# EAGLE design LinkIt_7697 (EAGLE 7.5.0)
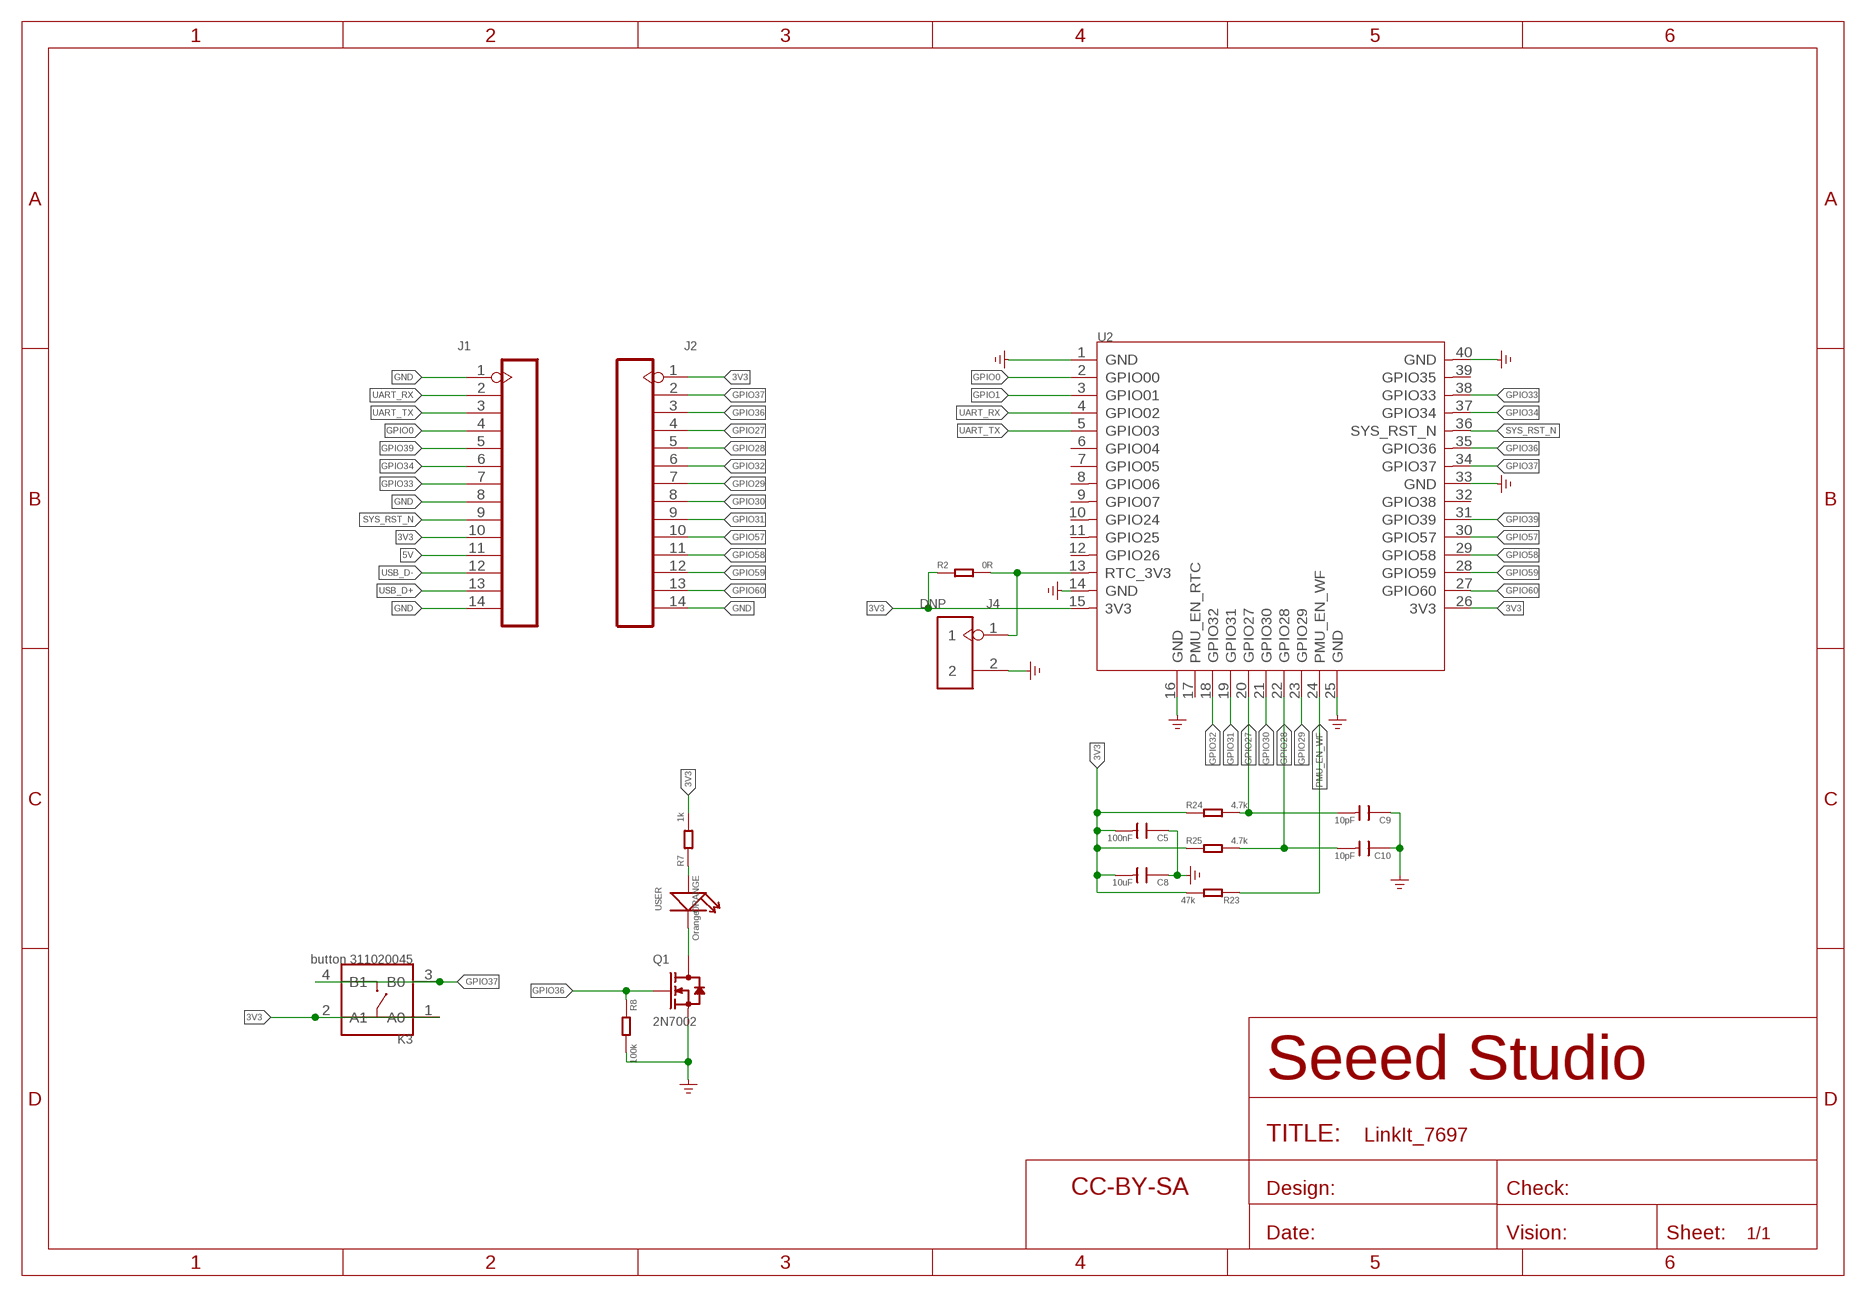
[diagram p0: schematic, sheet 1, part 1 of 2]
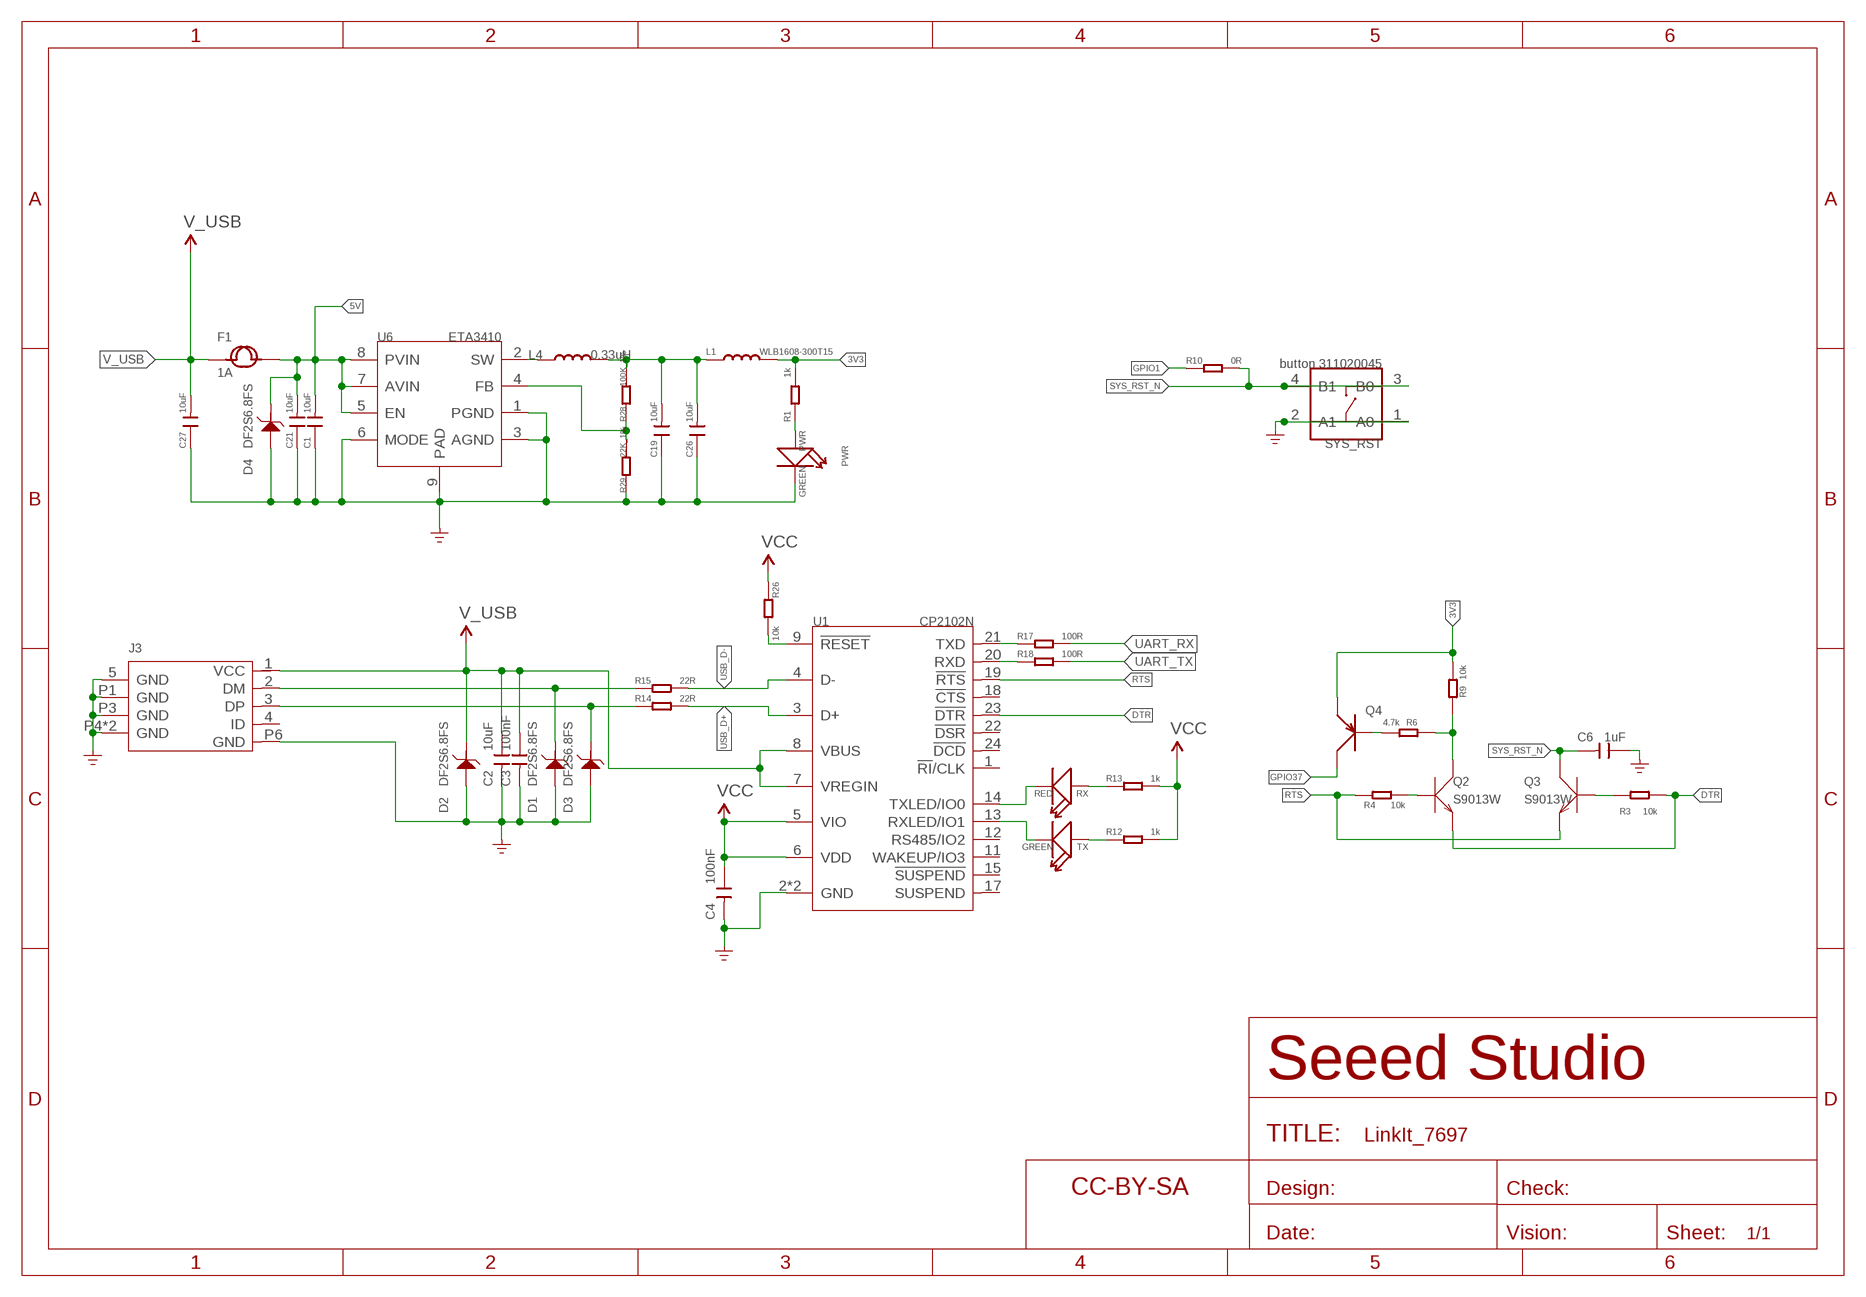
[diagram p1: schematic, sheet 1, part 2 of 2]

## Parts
C1  10uF  C-0402  [C0402]
C2  10uF  C-0402  [C0402]
C3  100nF  C-0402  [C0402]
C4  100nF  C-0402  [C0402]
C5  100nF  C-0402  [C0402]
C6  1uF  C-0402  [C0402]
C8  10uF  C-0402  [C0402]
C9  10pF  C-0402  [C0402]
C10  10pF  C-0402  [C0402]
C19  10uF  C-0402  [C0402]
C21  10uF  C-0402  [C0402]
C26  10uF  C-0402  [C0402]
C27  10uF  C-0402  [C0402]
D1  DF2S6.8FS  D-ESD-2P'DF2S6.8FS'  [SOD-923]
D2  DF2S6.8FS  D-ESD-2P'DF2S6.8FS'  [SOD-923]
D3  DF2S6.8FS  D-ESD-2P'DF2S6.8FS'  [SOD-923]
D4  DF2S6.8FS  D-ESD-2P'DF2S6.8FS'  [SOD-923]
F1  1A  FUSE'1206'  [F1206]
FR1  SEEEDSTUDIO-OPEN-SCH-FRAME  [SEEEDSTUDIO-PCB-FRAME]
FR2  SEEEDSTUDIO-OPEN-SCH-FRAME  [SEEEDSTUDIO-PCB-FRAME]
J1  HEADER-14P-2.54  [H14-2.54]
J2  HEADER-14P-2.54  [H14-2.54]
J3  MICRO-USB5+4P  [MICRO-USB5+5P-SMD-0.65-7.2X5.06MM]
J4  DNP  HEADER-2P-2.0  [H2-2.0-C55D32MIL]
K3  button 311020045  BUTTON-4P-4.5X3.2  [SW4P-SMD-4.5X3.2X2.5MM]
L1  WLB1608-300T15  L-0603  [L0603]
L4  0.33uH  L-MPM201610SR33_T  [L201610]
ORANGE  Orange  LED'0603'  [LED-0603]
PWR  GREEN  LED'0603'  [LED-0603]
Q1  2N7002  MOSFET-N'SI1304BDL'  [SOT-323]
Q2  S9013W  TRANSISTOR-NPN-SOT323  [SOT-323]
Q3  S9013W  TRANSISTOR-NPN-SOT323  [SOT-323]
Q4  TRANSISTOR-PNP  [SOT-323]
R1  1k  R-0402  [R0402]
R2  0R  R-0603  [R0603]
R3  10k  R-0402  [R0402]
R4  10k  R-0402  [R0402]
R6  4.7k  R-0402  [R0402]
R7  1k  R-0402  [R0402]
R8  100k  R-0402  [R0402]
R9  10k  R-0402  [R0402]
R10  0R  R-0402  [R0402]
R12  1k  R-0402  [R0402]
R13  1k  R-0402  [R0402]
R14  22R  R-0402  [R0402]
R15  22R  R-0402  [R0402]
R17  100R  R-0402  [R0402]
R18  100R  R-0402  [R0402]
R23  47k  R-0402  [R0402]
R24  4.7k  R-0402  [R0402]
R25  4.7k  R-0402  [R0402]
R26  10k  R-0402  [R0402]
R28  100K_1%  R-0402  [R0402]
R29  22K_1%  R-0402  [R0402]
RX  RED  LED'0603'  [LED-0603]
SYS_RST  button 311020045  BUTTON-4P-4.5X3.2  [SW4P-SMD-4.5X3.2X2.5MM]
TX  GREEN  LED'0603'  [LED-0603]
U1  CP2102N  CONVERTER-CP2102N(QFN24)  [QFN24G-0.5-4X4MM]
U2  MOUDLE-MT7697F  [MOUDLE40P-1.27-22X18MM]
U6  ETA3410  CONVERTER-ETA3410  [DFN8G-0.5-2X2MM]

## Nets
3V3: C5.2 C8.2 J1.10 J2.1 K3.1(A0) K3.2(A1) L1.2 Q4.2(E) R1.2 R2.1 R7.2 R9.1 R23.2 R24.1 R25.1 U2.15(3V3) U2.26(3V3)
5V: C1.2 C21.2 D4.1 F1.2 J1.11 U6.5(EN) U6.7(AVIN) U6.8(PVIN)
D-: D1.1 J3.2(DM) R15.1
DTR: Q2.2(E) R3.1 U1.23(!DTR!)
GND: C1.1 C2.2 C3.2 C4.2 C5.1 C6.1 C8.1 C9.1 C10.1 C19.1 C21.1 C26.1 C27.1 D1.2 D2.2 D3.2 D4.2 J1.1 J1.8 J1.14 J2.14 J3.5(GND) J3.P1(GND) J3.P3(GND) J3.P4(GND) J3.P5(GND) J3.P6(GND) J4.2 PWR.- Q1.2(S) R8.2 R29.1 SYS_RST.1(A0) SYS_RST.2(A1) U1.2(GND) U1.PAD(GND) U2.1(GND) U2.14(GND) U2.16(GND) U2.25(GND) U2.33(GND) U2.40(GND) U6.1(PGND) U6.3(AGND) U6.6(MODE) U6.9(PAD) ; supply symbol labelled GND_POWER
GPIO0: J1.4 U2.2(GPIO00)
GPIO1: R10.1 U2.3(GPIO01)
GPIO27: C9.2 J2.4 R24.2 U2.20(GPIO27)
GPIO28: C10.2 J2.5 R25.2 U2.22(GPIO28)
GPIO29: J2.7 U2.23(GPIO29)
GPIO30: J2.8 U2.21(GPIO30)
GPIO31: J2.9 U2.19(GPIO31)
GPIO32: J2.6 U2.18(GPIO32)
GPIO33: J1.7 U2.38(GPIO33)
GPIO34: J1.6 U2.37(GPIO34)
GPIO36: J2.3 Q1.1(G) R8.1 U2.35(GPIO36)
GPIO37: J2.2 K3.3(B0) K3.4(B1) Q4.3(C) U2.34(GPIO37)
GPIO39: J1.5 U2.31(GPIO39)
GPIO57: J2.10 U2.30(GPIO57)
GPIO58: J2.11 U2.29(GPIO58)
GPIO59: J2.12 U2.28(GPIO59)
GPIO60: J2.13 U2.27(GPIO60)
N$1: J4.1 R2.2 U2.13(RTC_3V3)
N$2: C19.2 C26.2 L1.1 L4.2 R28.2
N$3: D3.1 J3.3(DP) R14.1
N$4: PWR.+ R1.1
N$5: Q4.1(B) R6.1
N$6: ORANGE.+ R7.1
N$7: Q3.1(B) R3.2
N$8: ORANGE.- Q1.3(D)
N$9: Q2.1(B) R4.2
N$10: TX.- U1.13(RXLED/IO1)
N$11: Q2.3(C) R6.2 R9.2
N$13: RX.- U1.14(TXLED/IO0)
N$15: R26.2 U1.9(!RESET!)
N$17: R18.1 U1.20(RXD)
N$18: R17.1 U1.21(TXD)
N$29: L4.1 U6.2(SW)
N$32: R28.1 R29.2 U6.4(FB)
N$36: R12.1 TX.+
N$37: R13.1 RX.+
PMU_EN_WF: R23.1 U2.24(PMU_EN_WF)
RTS: Q3.2(E) R4.1 U1.19(!RTS!)
SYS_RST_N: C6.2 J1.9 Q3.3(C) R10.2 SYS_RST.3(B0) SYS_RST.4(B1) U2.36(SYS_RST_N)
UART_RX: J1.2 R17.2 U2.4(GPIO02)
UART_TX: J1.3 R18.2 U2.5(GPIO03)
USB_D+: J1.13 R14.2 U1.3(D+)
USB_D-: J1.12 R15.2 U1.4(D-)
V_USB: C2.1 C3.1 C27.2 D2.1 F1.1 J3.1(VCC) U1.7(VREGIN) U1.8(VBUS)
VCC: C4.1 R12.2 R13.2 R26.1 U1.5(VIO) U1.6(VDD)
Unconnected: J3.4(ID) U1.1(!RI!/CLK) U1.11(WAKEUP/IO3) U1.12(RS485/IO2) U1.15(!SUSPEND!) U1.17(SUSPEND) U1.18(!CTS!) U1.22(!DSR!) U1.24(!DCD!) U2.6(GPIO04) U2.7(GPIO05) U2.8(GPIO06) U2.9(GPIO07) U2.10(GPIO24) U2.11(GPIO25) U2.12(GPIO26) U2.17(PMU_EN_RTC) U2.32(GPIO38) U2.39(GPIO35)

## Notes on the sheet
- PWR
- USER

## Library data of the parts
C1-C6 C8-C10 C19 C21 C26 C27 = Discrete-small:C*: Ceramic Capacitors
D1-D4 = Discrete-new:D-ESD-2P: SOD-923:304060009;SOD-123:304060001
F1 = C-R-package test:FUSE
FR1 FR2 = moudle-new:SEEEDSTUDIO-OPEN-SCH-FRAME
J1 J2 = Connector-new:HEADER-14P: Header 14 Standard 14-pin 0.1" header. Use with straight break away headers (SKU : PRT-00116), right angle break away headers (PRT-00553), swiss pins (PRT-00743), machine pins (PRT-00117), and female headers (PRT-00115).
J3 = Connector-new:MICRO-USB5+4P: 5+4P-SMD-0.65-B:320010000;5+2P-SMD-0.65-AB:340032001;5+5P-SMD-0.65-7.2X5.06MM:320010050;
J4 = Connector-new:HEADER-2P
K3 SYS_RST = Discrete-new:BUTTON-4P: SW4-6.0X6.0X5.0MM:311020024;SW4-8.0X8.0X9.0MM:311020028;SW4-SMD-6.0X6.0X5.0MM:311020004;SW4-SMD-3.35X3.35X1.5MM:311020030;SW4-SMD-5.2X5.2X2.5MM:311020046
L1 = Discrete-small:L
L4 = Discrete-new:L
ORANGE PWR RX TX = Discrete-small:LED
Q1 = Discrete-new:MOSFET-N
Q2 Q3 = Discrete-new:TRANSISTOR-NPN: NPN audion
Q4 = Discrete-new:TRANSISTOR-PNP: PNP audion
R1-R4 R6-R10 R12-R15 R17 R18 R23-R26 R28 R29 = Discrete-small:R*
U1 = template:CONVERTER-CP2102N(QFN24)
U2 = template:MOUDLE-MT7697F
U6 = template:CONVERTER-ETA3410: 3MHZ 2A High Step-Down Converter in DFN2x2-8L Package

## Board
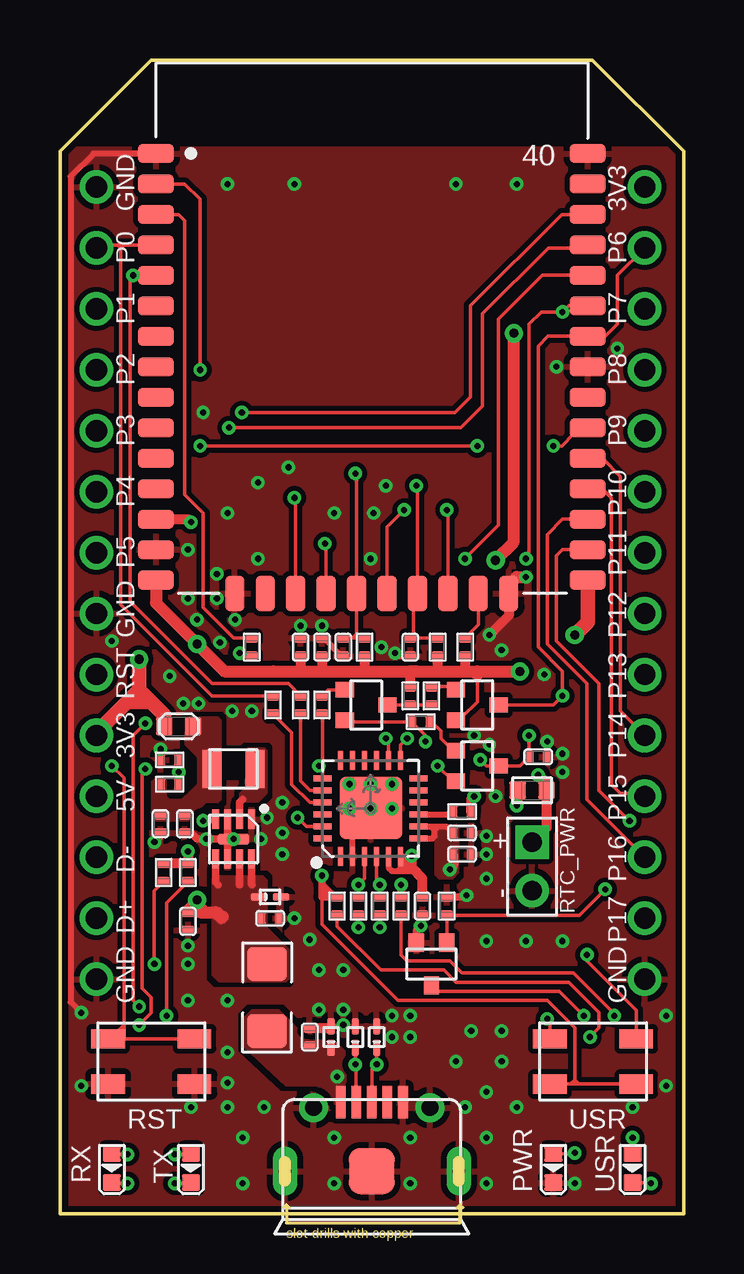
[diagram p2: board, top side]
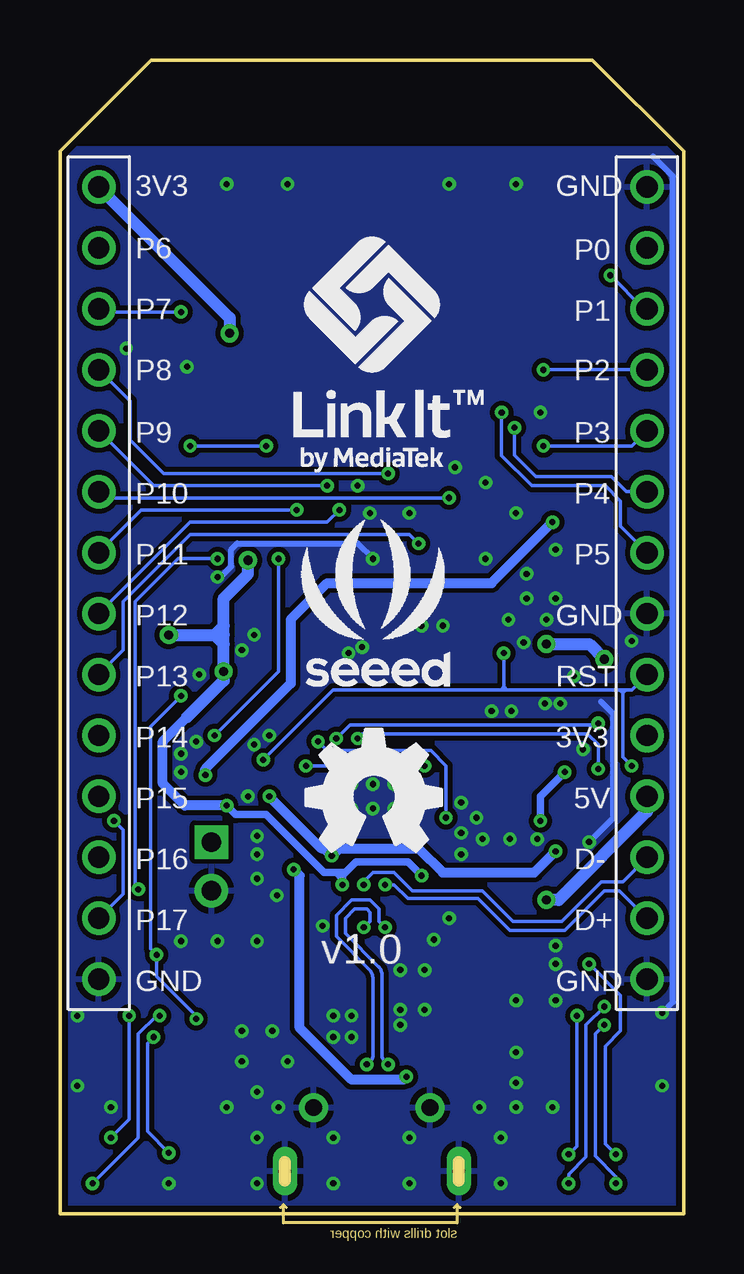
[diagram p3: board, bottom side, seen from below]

Size 26 x 48.09 mm. Coordinates in mm from the lower left corner, seen from the top.
Outline: 0,0 26,0 26,44.28 22.19,48.09 3.81,48.09 0,44.28 0,0
Copper layers (1*16): Top 0.035mm / dielectric 1.5mm / Bottom 0.035mm
Design rules "SeeedStudio_2layer_DRU_no_angle_20140221 *": minimum track width 1mil, minimum drill 10mil, track to track 6mil, track to pad 6mil, pad to pad 6mil, via to via 6mil, smd to smd 0mil, copper to edge 10mil, drill to drill 10mil, minimum pad ring 10mil, minimum via ring 6mil, stop-mask expansion 2mil, vias tented up to drill 25mil, thermal gap 10mil
tRestrict: area 0,44.7 to 26,48.3; area 7,18.3 to 7.5,19.3
bRestrict: area 0,44.7 to 26,48.3

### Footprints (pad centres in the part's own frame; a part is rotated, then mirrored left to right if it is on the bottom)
C0402 = smd 0.508 x 0.385: 1 0,0.383; 2 0,-0.383
SOD-923 = smd 0.7 x 0.3: 1 -0.45,0; 2 0.45,0
F1206 = smd 1.397 x 1.651: 1 -1.397,0; 2 1.397,0
H14-2.54 = drill 0.889 pad 1.397: 1 0,-16.51; 2 0,-13.97; 3 0,-11.43; 4 0,-8.89; 5 0,-6.35; 6 0,-3.81; 7 0,-1.27; 8 0,1.27; 9 0,3.81; 10 0,6.35; 11 0,8.89; 12 0,11.43; 13 0,13.97; 14 0,16.51
MICRO-USB5+5P-SMD-0.65-7.2X5.06MM = smd 0.4 x 1.35: 1 -1.3,2.875; 2 -0.65,2.875; 3 0,2.875; 4 0.65,2.875; 5 1.3,2.875 | smd 1.9 x 1.9: P1 0,0 | drill 0.508 pad 1.016 long: P3 -3.625,0; P4 3.625,0 | drill 0.7: P5 -2.425,2.65; P6 2.425,2.65
H2-2.0-C55D32MIL = drill 0.813 pad 1.397 square: 1 -1.016,0 | drill 0.813 pad 1.397: 2 1.016,0
SW4P-SMD-4.5X3.2X2.5MM = smd 1.4 x 0.8: 1 -1.8,-0.94; 2 1.8,-0.94; 3 1.8,0.94; 4 -1.8,0.94
L0603 = smd 0.762 x 0.696: 1 0,0.602; 2 0,-0.602
L201610 = smd 0.8 x 1.6: 1 -0.9,0; 2 0.9,0
LED-0603 = smd 0.696 x 0.762: + -0.602,0; - 0.602,0
SOT-323 = smd 0.635 x 0.762: 1 -0.635,-0.889; 2 0.635,-0.889; 3 0,0.889
R0402 = smd 0.508 x 0.385: 1 0,0.383; 2 0,-0.383
R0603 = smd 0.762 x 0.696: 1 0,0.602; 2 0,-0.602
QFN24G-0.5-4X4MM = smd 0.8 x 0.26: 1 -2,1.25; 2 -2,0.75; 3 -2,0.25; 4 -2,-0.25; 5 -2,-0.75; 6 -2,-1.25; 13 2,-1.25; 14 2,-0.75; 15 2,-0.25; 16 2,0.25; 17 2,0.75; 18 2,1.25 | smd 0.26 x 0.8: 7 -1.25,-2; 8 -0.75,-2; 9 -0.25,-2; 10 0.25,-2; 11 0.75,-2; 12 1.25,-2; 19 1.25,2; 20 0.75,2; 21 0.25,2; 22 -0.25,2; 23 -0.75,2; 24 -1.25,2 | smd 2.6 x 2.6: PAD 0.02,-0.01
MOUDLE40P-1.27-22X18MM = smd 1.5 x 0.8: 1 -9,8.89; 2 -9,7.62; 3 -9,6.35; 4 -9,5.08; 5 -9,3.81; 6 -9,2.54; 7 -9,1.27; 8 -9,0; 9 -9,-1.27; 10 -9,-2.54; 11 -9,-3.81; 12 -9,-5.08; 13 -9,-6.35; 14 -9,-7.62; 15 -9,-8.89; 26 9,-8.89; 27 9,-7.62; 28 9,-6.35; 29 9,-5.08; 30 9,-3.81; 31 9,-2.54; 32 9,-1.27; 33 9,0; 34 9,1.27; 35 9,2.54; 36 9,3.81; 37 9,5.08; 38 9,6.35; 39 9,7.62; 40 9,8.89 | smd 0.8 x 1.5: 16 -5.715,-9.45; 17 -4.445,-9.45; 18 -3.175,-9.45; 19 -1.905,-9.45; 20 -0.635,-9.45; 21 0.635,-9.45; 22 1.905,-9.45; 23 3.175,-9.45; 24 4.445,-9.45; 25 5.715,-9.45
DFN8G-0.5-2X2MM = smd 0.8 x 0.3: 1 -0.827,0.75; 2 -0.827,0.25; 3 -0.827,-0.25; 4 -0.827,-0.75; 5 0.827,-0.75; 6 0.827,-0.25; 7 0.827,0.25; 8 0.827,0.75 | smd 0.45 x 1.3: 9 0,0

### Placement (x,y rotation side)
C1  5.33,12.19 180 top
C2  16.76,14.99 90 top
C3  16.76,15.88 90 top
C4  15.11,12.83 0 top
C5  10.03,23.62 0 top
C6  19.94,19.05 270 top
C8  10.92,23.62 0 top
C9  11.81,23.62 180 top
C10  14.61,23.62 180 top
C19  5.21,16.26 180 top
C21  8.76,12.32 270 top
C26  4.19,16.26 180 top
C27  10.41,7.37 0 top
D1  12.32,7.37 90 top
D2  11.3,7.37 90 top
D3  13.21,7.37 90 top
D4  8.76,13.21 0 top
F1  8.64,9.02 90 top
FR1  not placed on the board
FR2  not placed on the board
J1  1.52,26.29 180 bottom
J2  24.38,26.29 180 bottom
J3  13,1.78 0 top
J4  19.68,14.48 270 top
K3  22.23,6.35 0 top
L1  4.95,20.32 270 top
L4  7.24,18.54 180 top
ORANGE  23.88,1.91 270 top
PWR  20.57,1.91 270 top
Q1  15.49,10.41 180 top
Q2  12.76,21.21 270 top
Q3  17.4,18.67 270 top
Q4  17.4,21.21 270 top
R1  11.56,12.83 180 top
R2  19.68,17.65 90 top
R3  15.05,20.51 90 top
R4  10.92,21.21 180 top
R6  15.49,21.59 0 top
R7  14.22,12.83 180 top
R8  16.13,12.83 180 top
R9  14.61,21.59 0 top
R10  8,23.62 0 top
R12  5.33,14.22 180 top
R13  4.32,14.22 180 top
R14  12.45,12.83 180 top
R15  13.34,12.83 180 top
R17  8.89,21.21 180 top
R18  10.03,21.21 180 top
R23  16.89,23.62 0 top
R24  12.7,23.62 180 top
R25  15.75,23.62 180 top
R26  16.76,16.76 270 top
R28  4.57,17.91 270 top
R29  4.57,18.92 90 top
RX  2.16,1.91 270 top
SYS_RST  3.81,6.35 0 top
TX  5.46,1.91 270 top
U1  12.95,16.89 90 top
U2  13,35.31 0 top
U6  7.24,15.62 270 top
U$1  [OSHW_FILLX200_NOTEXT_TNAME]  15.75,15.11 0 bottom
U$3  [SEEED-SILK-TNAME-280*268MIL]  12.95,25.65 0 bottom

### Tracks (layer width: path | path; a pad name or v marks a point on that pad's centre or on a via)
3V3  (via drill 0.25 pad 0.51, 0.38 pad 0.76)
  Top 0.152: K3.2 21.64,5.41 | 21.64,5.41 21.46,5.41 | 21.46,5.41 21.29,5.41 | 21.29,5.41 K3.1 | 21.46,5.59 21.46,7.75 20.32,8.89 14.1,8.89 10.92,12.06 10.92,13.21 | 21.46,5.59 21.46,5.41 | 21.29,5.41 21.46,5.59 | 21.64,5.41 21.46,5.59 | 17.4,22.23 17.4,21.34 16.76,20.7 16.76,20.57 Q4.2 | 17.4,22.23 17.4,22.61 | 17.4,22.23 17.14,22.48 | 17.4,22.23 17.65,22.48
  Top 0.305: R7.2 v14.22,13.72 | v10.92,14.1 10.92,13.72 | 10.92,13.72 10.92,13.21 R1.2 11.43,13.21 10.92,13.72
  Top 0.406: C5.2 10.03,22.61 | C8.2 10.92,22.61 | R24.1 12.7,22.61 | R25.1 15.75,22.61 | R23.2 16.89,22.61 | 14.73,22.6 14.73,22.61 | 19.08,17.81 R2.1 19.08,17.05 v19.05,17.02 | R9.1 14.61,22.61 14.86,22.61
  Top 0.508: U2.15 4,25.46 v5.71,23.75 6.86,22.61 8.89,22.61 10.03,22.61 10.92,22.61 12.7,22.61 14.61,22.61 14.73,22.61 14.86,22.61 15.75,22.61 16.89,22.61 17.4,22.61 v19.18,22.61 | v18.16,27.24 18.92,28 v18.92,36.7
  Top 0.61: J1.10 1.52,20.07 2.79,21.34 | U2.26 22,24.67 v21.46,24.13 | L1.2 4.35,20.8 3.81,21.34 | 3.81,21.34 3.17,21.34 | 3.17,21.34 2.79,21.34 | v3.3,23.11 3.3,21.84 | 3.3,21.84 3.3,21.46 3.17,21.34 | 3.3,21.84 2.79,21.34 | 3.3,21.84 3.81,21.34
  Bottom 0.305: 14.48,14.22 14.99,14.22 17.4,16.64 18.67,16.64 v19.05,17.02 | 14.48,14.22 14.22,14.22 | 14.22,14.22 14.1,14.22 | 14.1,14.22 13.65,14.67 11.49,14.67 v10.92,14.1 | 14.22,14.1 14.22,14.22 | 14.22,13.97 14.22,14.1 | 14.22,14.1 14.1,14.22 | v14.22,13.72 14.22,13.97 | 14.22,13.97 14.48,14.22
  Bottom 0.406: v19.05,17.02 20.8,17.02 21.72,17.93 21.72,19.68 20.7,20.7
  Bottom 0.508: J2.1 18.92,37.34 v18.92,36.7 | v5.71,23.75 3.94,23.75 v3.3,23.11 | v18.16,27.24 18.16,26.67 19.18,25.65 19.18,24.51 | 20.7,20.7 19.18,22.23 v19.18,22.61 19.18,23.75 | 19.18,24.13 19.18,24.51 | v21.46,24.13 19.56,24.13 | 19.56,24.13 19.18,24.13 | 19.56,24.13 19.18,24.51 | 19.56,24.13 19.18,23.75 | 19.18,23.75 19.18,24.13
5V  (via drill 0.38 pad 0.76)
  Top 0.305: U6.5 6.49,13.83 6.6,13.72 | U6.7 7.49,13.72 | U6.8 7.99,13.73 8,13.72
  Top 0.406: 6.6,12.57 6.79,12.38 | 5.84,12.57 C1.2 5.33,12.7 v5.71,13.08 5.71,12.95 5.97,12.7
  Top 0.508: 5.84,12.57 6.48,12.57 6.73,12.32 6.79,12.38
  Bottom 0.508: J1.11 1.52,16.76 5.21,13.08 v5.71,13.08
  pour Top (isolate 0.254, no thermals): 6.48,14.1 8.46,14.1 8.64,13.92 8.64,11.94 9.53,11.05 9.53,9.78 9.4,9.65 6.63,9.65 6.35,9.94 6.35,13.97
D-  (via drill 0.25 pad 0.51)
  Top 0.152: R15.1 v13.34,11.94 | D1.1 v12.32,6.22 12.35,6.19 J3.2
  Bottom 0.152: v13.34,11.94 13.08,12.19 13.08,12.57 13.21,12.7 13.72,12.7 14.1,12.32 14.1,11.68 12.73,10.32 arc45 12.57,9.94 12.57,6.6 arc-45 12.49,6.39 v12.32,6.22
DTR  (via drill 0.25 pad 0.51)
  Top 0.152: U1.23 10.28,16.14 v9.91,16.51 | v15.24,19.68 15.24,19.94 R3.1 11.94,20.51 Q2.2
  Bottom 0.152: v9.91,16.51 9.91,18.67 10.54,19.3 14.86,19.3 v15.24,19.68
GND  (via drill 0.25 pad 0.51)
  Top 0.254: C9.1 11.75,23.24 10.98,24 C8.1 | U1.2 12.2,16.75 v12.06,16.89 | C10.1 14.1,23.24 v13.97,23.37 | v0.89,8.38 0.45,8.83 0.45,43.24 1.4,44.2 U2.1
  Top 0.305: U6.6 6.99,15.37 U6.9 | U6.3 6.99,15.87 U6.9 | C19.1 5.46,15.87 5.71,15.62 v6.1,15.62 U6.9 | R8.2 16.89,13.21 v16.95,13.27 | C4.2 15.11,12.06 v15.05,12 14.86,11.81 Q1.2 | R29.1 v4.19,19.37 | C26.1 4.19,15.75 v3.94,15.49
  Top 0.406: U2.25 18.71,24.94 v17.91,24.13 | C27.1 11.24,7.75 D2.2
  Top 0.508: U2.25 18.71,26.21 19.05,26.54 v19.43,26.54
  Bottom 0.254: v0.89,8.38 0.45,8.83 0.45,43.24 1.27,44.07 | v3.94,15.49 2.92,16.51 2.92,20.83 3.43,21.34 | v19.43,26.54 19.3,26.54 18.86,26.99 18.86,27.69 18.61,27.94 13.59,27.94 v12.95,27.3
  other vias: 7.24,15.62 8.38,15.62 10.92,24.51 10.03,24.51 19.05,42.93 12.95,16.89 13.84,16.89 12.06,17.91 12.95,17.91 13.84,17.91 17.78,15.75 17.78,14.99 20.95,11.37 17.78,13.97 13.4,23.62 8.64,16.51 8.26,27.3 8.26,30.48 6.99,42.93 9.78,42.93 16.51,42.93 8.51,4.45 5.46,4.45 0.89,5.33 17.78,1.27 23.88,4.45 25.27,8.26 7.62,3.17 25.27,5.33 17.78,11.37 16.89,4.45 17.78,3.17 19.43,11.37 5.78,21.27 5.14,21.27 21.46,1.27 19.05,4.45 7.62,1.27 20.95,18.41 9.27,14.99 5.33,11.18 5.33,10.41 10.79,8.51 10.79,10.16 11.81,8.51 13.84,8.26 14.61,8.26 14.61,7.37 9.27,17.14 11.81,7.87 13.84,7.37 18.16,17.4 9.27,15.88 5.33,8.89 6.99,8.89 11.81,10.16 2.16,23.88 8,20.95 6.99,4.45 6.99,5.46 6.99,6.73 6.99,29.21 20.7,35.31 13.59,30.35 13.08,29.21 11.43,29.21 23.24,36.07 5.97,33.4 9.53,31.11 14.61,3.17 14.61,1.27 11.43,1.27 11.43,3.17 20.95,19.18 5.33,27.69 5.33,25.65 6.54,25.65 6.54,26.67 9.78,12.32 10.41,11.43 7.18,20.95 7.3,24.77 5.71,24.77 4.57,22.42 6.67,23.81 18.41,23.5 20.19,22.48 17.14,7.62 18.41,7.62 18.41,6.35 16.51,6.35 17.78,5.08 17.27,19.94 17.91,19.56 20.32,19.68
  pour Bottom (isolate 0.203, rank 6): -0.64,48.9 26.67,48.9 26.67,-0.64 -0.64,-0.64
  pour Top (isolate 0.203, rank 6): -0.64,48.9 26.67,48.9 26.67,-0.64 -0.64,-0.64
GPIO0  (via drill 0.25 pad 0.51)
  Top 0.152: U2.2 5.21,42.93 5.84,42.29 v5.84,35.18
  Bottom 0.152: J1.4 v5.84,35.18
GPIO1
  Top 0.152: U2.3 4.95,41.66 5.21,41.4 5.21,29.97 5.97,29.21 5.97,25.27 7.24,24 R10.1
GPIO27  (via drill 0.25 pad 0.51)
  Top 0.152: C9.2 12.32,24 | 12.32,24 R24.2 | 12.37,24.18 U2.20 12.37,30.82 v12.32,30.86 | 12.37,24.18 12.37,24.05 12.32,24 | 12.37,24.18 12.19,24 | 12.37,24.18 12.4,24.18 12.57,24
  Bottom 0.152: J2.4 23.08,33.87 23.08,32.26 21.68,30.86 v12.32,30.86
GPIO28  (via drill 0.25 pad 0.51)
  Top 0.152: v14.86,30.35 14.9,30.31 U2.22 14.73,25.68 14.73,24 C10.2 R25.2
  Bottom 0.152: v14.86,30.35 22.1,30.35 J2.5
GPIO29  (via drill 0.25 pad 0.51)
  Top 0.152: U2.23 16.18,29.29 v16.13,29.34
  Bottom 0.152: J2.7 22.61,29.34 v16.13,29.34
GPIO30  (via drill 0.25 pad 0.51)
  Top 0.152: U2.21 13.63,28.62 v14.35,29.34
  Bottom 0.152: J2.8 20.57,28.83 14.86,28.83 v14.35,29.34
GPIO31  (via drill 0.25 pad 0.51)
  Top 0.152: U2.19 11.1,27.89 v11.05,27.94
  Bottom 0.152: v11.05,27.94 11.43,28.32 20.57,28.32 23.37,25.53 23.37,23.5 J2.9
GPIO32  (via drill 0.25 pad 0.51)
  Top 0.152: U2.18 9.82,29.8 v9.78,29.84
  Bottom 0.152: J2.6 24.13,29.84 v9.78,29.84
GPIO33  (via drill 0.25 pad 0.51)
  Top 0.152: 21.69,41.66 U2.38 20.92,41.66 17.11,37.85 17.11,34.04 16.48,33.4 v7.58,33.4
  Bottom 0.152: J1.7 2.63,28.67 2.63,29.72 3.27,30.35 6.33,30.35 7.58,31.61 v7.58,33.4
GPIO34  (via drill 0.25 pad 0.51)
  Top 0.152: 21.46,40.13 21.75,40.13 U2.37 21.87,40.26 20.36,40.26 17.62,37.52 17.62,33.66 16.72,32.77 v7.05,32.77
  Bottom 0.152: v7.05,32.77 7.05,31.63 6.15,30.73 3.01,30.73 2.38,30.1 J1.6
GPIO36  (via drill 0.25 pad 0.51)
  Top 0.152: Q1.1 R8.1 | R8.1 | R8.1 21.65,12.44 v22.73,13.53 | U2.35 21.21,37.85 v20.95,37.59 20.07,37.59 19.56,37.08 19.56,27.56 19.43,27.43 v19.43,27.3
  Bottom 0.152: v22.73,13.53 22.86,13.65 22.86,25.53 21.08,27.3 v19.43,27.3 | v20.95,37.59 24.26,37.59 J2.3
GPIO37  (via drill 0.25 pad 0.51)
  Top 0.152: J2.2 23.24,39.12 23.24,37.08 22.73,36.58 U2.34 20.34,36.58 19.94,36.17 19.94,23.62 20.95,22.61 v20.95,21.59 20.57,21.21 Q4.3 | K3.3 24.02,8.49 21.97,10.54 v21.97,10.79 | K3.4 20.43,8.02 v20.32,8.13
  Bottom 0.152: v20.32,8.13 20.32,8.26 21.97,9.91 v21.97,10.79 22.23,11.05 22.23,20.32 v20.95,21.59
GPIO39  (via drill 0.25 pad 0.51)
  Top 0.152: v17.4,32 v5.84,32 | v20.57,32 20.92,32 21.43,32.51 21.75,32.51 U2.31
  Bottom 0.152: v17.4,32 v20.57,32 | v5.84,32 2.16,32 J1.5
GPIO57
  Top 0.152: U2.30 22.61,31.5 23.37,30.73 23.37,20.95 J2.10
GPIO58
  Top 0.152: U2.29 22.61,30.23 22.99,29.84 22.99,17.91 23.37,17.53 24.26,17.53 J2.11
GPIO59
  Top 0.152: U2.28 20.95,28.96 20.32,28.32 20.32,23.75 21.97,22.1 21.97,17.27 J2.12
GPIO60  (via drill 0.25 pad 0.51)
  Top 0.152: U2.27 20.95,27.69 20.7,27.43 20.7,23.88 22.48,22.1 22.48,17.65 v23.75,16.38
  Bottom 0.152: J2.13 23.37,13.34 23.37,16 v23.75,16.38
N$1  (via drill 0.25 pad 0.51)
  Top 0.406: J4.1 20.29,16.1 R2.2 20.29,17.94 v19.94,18.29 | U2.13 5.33,28.96 v5.46,28.83
  Bottom 0.406: v19.94,18.29 19.94,18.54 16.38,22.1 16.38,24.77 14.86,26.29 8,26.29 v5.46,28.83
N$2
  pour Top (isolate 0.254, no thermals): 4.32,18.16 3.94,18.16 3.81,18.03 3.81,16.51 3.94,16.38 5.33,16.38 6.1,17.14 6.6,17.14 6.73,17.27 6.73,20.57 6.6,20.7 5.39,20.7 5.21,20.52 5.21,19.56 5.71,19.05 5.71,17.91 5.08,17.27 4.57,17.27 4.45,17.4 4.45,18.03
N$3  (via drill 0.25 pad 0.51)
  Top 0.152: R14.1 v12.45,11.94 | D3.1 v13.21,6.22 13,6.01 J3.3
  Bottom 0.152: v12.45,11.94 12.7,12.19 12.7,12.7 13.08,13.08 13.84,13.08 14.48,12.45 14.48,11.56 13.11,10.19 arc45 12.95,9.81 12.95,6.58 arc45 13.03,6.4 v13.21,6.22
N$4  (via drill 0.25 pad 0.51)
  Top 0.152: R1.1 11.56,11.98 13.38,10.16 16,10.16 16.51,9.65 21.22,9.65 22.48,8.39 22.48,7.75 v22.1,7.37 | PWR.+ 21.43,2.51 v21.46,2.54
  Bottom 0.152: v22.1,7.37 22.35,7.11 22.35,3.43 v21.46,2.54
N$5
  Top 0.152: Q4.1 16.38,21.97 R6.1
N$6  (via drill 0.25 pad 0.51)
  Top 0.152: R7.1 14.22,10.79 14.48,10.54 16.26,10.54 16.76,10.03 21.41,10.03 23.11,8.32 v23.11,8.26 | ORANGE.+ v23.88,3.17
  Bottom 0.152: v23.88,3.17 23.11,3.94 v23.11,8.26
N$7
  Top 0.152: Q3.1 16.38,19.3 15.88,19.81 15.88,20.13 15.5,20.51 R3.2
N$8  (via drill 0.25 pad 0.51)
  Top 0.152: ORANGE.- 24.61,1.3 v24.64,1.27 | Q1.3 15.75,9.27 20.83,9.27 v21.84,8.26
  Bottom 0.152: v24.64,1.27 22.73,3.17 22.73,7.5 21.97,8.26 v21.84,8.26
N$9
  Top 0.152: Q2.1 11.17,21.84 R4.2
N$10  (via drill 0.25 pad 0.51)
  Top 0.152: U1.13 14.2,19.54 v14.48,19.81 | v3.56,20.45 3.05,19.94 3.05,8.89 v3.3,8.64 | 5.3,1.28 5.32,1.3 TX.- 5.43,1.27 v4.79,1.27
  Bottom 0.152: v14.48,19.81 13.91,20.38 3.62,20.38 v3.56,20.45 | v3.3,8.64 4.06,7.87 4.06,2.38 4.79,1.65 v4.79,1.27
N$11
  Top 0.152: R6.2 R9.2 Q2.3
N$13  (via drill 0.25 pad 0.51)
  Top 0.152: v3.56,18.54 3.43,18.41 3.43,9.4 3.81,9.02 3.81,8.38 v3.3,7.87 | U1.14 13.7,19.7 v13.59,19.81 | RX.- 2.19,1.27 v2.82,1.27
  Bottom 0.152: v3.56,18.54 3.56,19.56 4,20 13.4,20 v13.59,19.81 | v3.3,7.87 3.68,7.49 3.68,2.41 2.82,1.55 v2.82,1.27
N$15
  Top 0.254: U1.9 16.26,16.64 R26.2
N$17
  Top 0.152: U1.20 10.43,17.64 10.03,18.03 R18.1
N$18
  Top 0.152: U1.21 10.42,17.14 9.65,17.91 9.65,20.07 9.4,20.32 R17.1
N$29
  Top 0.305: U6.2 7.49,17.14 7.62,17.27
  pour Top (isolate 0.254, no thermals): 7.87,19.43 8.51,19.43 8.64,19.3 8.64,17.53 8.26,17.14 7.62,17.14 7.49,17.27 7.49,17.53 7.75,17.78 7.75,19.3
N$32  (via drill 0.25 pad 0.51)
  Top 0.305: U6.4 6.03,16.45 v5.97,16.38 | R28.1 v4.95,18.41 v4.96,18.42 R29.2
  Bottom 0.305: v5.97,16.38 5.97,17.4 v4.95,18.41
N$36  (via drill 0.25 pad 0.51)
  Top 0.152: R12.1 4.45,12.95 v4.45,8.26 | v4.79,2.48 5.43,2.48 TX.+
  Bottom 0.152: v4.45,8.26 4.45,2.82 v4.79,2.48
N$37  (via drill 0.25 pad 0.51)
  Top 0.152: R13.1 3.94,13.46 v3.94,10.41 | RX.+ 2.19,2.48 v2.82,2.48
  Bottom 0.152: v3.94,10.41 2.63,9.11 2.63,7.62 3.27,6.99 3.27,2.92 v2.82,2.48
PMU_EN_WF
  Top 0.152: U2.24 17.45,24.56 R23.1
RTS  (via drill 0.25 pad 0.51)
  Top 0.152: R4.1 10.95,20.79 10.95,18.83 v10.79,18.67 10.95,18.51 U1.19 | Q3.2 16.38,18.03 v15.75,18.67
  Bottom 0.152: v10.79,18.67 v15.75,18.67
SYS_RST_N  (via drill 0.25 pad 0.51)
  Top 0.152: 2.67,7.87 2.67,18.16 v2.16,18.67 | 2.67,7.87 2.67,7.29 | SYS_RST.3 2.67,7.29 | 2.67,7.29 SYS_RST.4 | 2.67,7.87 2.29,7.49 | v17.53,18.92 17.78,18.67 Q3.3 19.18,18.67 C6.2 v19.56,19.94 | R10.2 7.62,23.24 v7.49,23.37 | U2.36 20.11,39.12 18.29,37.3 18.29,28.7 v16.89,27.3
  Bottom 0.152: v2.16,18.67 2.54,19.05 2.54,21.72 | v17.53,18.92 14.61,21.84 7.62,21.84 | J1.9 2.16,21.84 2.41,21.84 | 2.54,21.72 2.54,21.84 | 2.41,21.84 2.54,21.84 | 2.54,21.84 2.67,21.84 | 2.67,21.84 7.37,21.84 | 7.37,21.84 7.49,21.84 | 7.49,21.84 7.62,21.84 | 2.54,21.72 2.41,21.84 | 2.54,21.72 2.67,21.84 | v7.49,23.37 7.49,21.97 | 7.49,21.97 7.49,21.84 | 7.37,21.84 7.49,21.97 | 7.49,21.97 7.62,21.84 | v16.89,27.3 16.89,22.61 v19.56,19.94
UART_RX
  Top 0.152: U2.4 2.67,40.39 | 2.67,40.39 2.54,40.39 | 2.54,40.39 2.41,40.39 | 2.41,40.39 1.65,40.39 J1.2 | 2.54,40.26 2.54,25.4 6.35,21.59 R17.2 | 2.54,40.26 2.54,40.39 | 2.54,40.26 2.41,40.39 | 2.54,40.26 2.67,40.39
UART_TX  (via drill 0.25 pad 0.51)
  Top 0.152: U2.5 v3.05,39.12 2.92,38.99 2.92,25.53 6.35,22.1 9.53,22.1 R18.2
  Bottom 0.152: J1.3 1.65,37.72 v3.05,39.12
USB_D+  (via drill 0.25 pad 0.51)
  Top 0.152: U1.3 12.7,13.97 v12.45,13.72 R14.2
  Bottom 0.152: v12.45,13.72 12.06,13.72 11.49,13.14 8.57,13.14 7.24,11.81 4.95,11.81 3.3,13.46 2.67,13.46 J1.13
USB_D-  (via drill 0.25 pad 0.51)
  Top 0.152: R15.2 v13.34,13.72 13.34,13.84 13.2,13.97 U1.4
  Bottom 0.152: J1.12 2.54,13.84 3.43,13.84 5.08,12.19 7.11,12.19 8.38,13.46 11.3,13.46 12.06,14.22 12.95,14.22 13.34,13.84 v13.34,13.72
V_USB  (via drill 0.25 pad 0.51)
  Top 0.254: U1.8 15.62,16.14 | 15.62,16.14 15.76,16.14 | 15.76,16.14 16.11,16.14 C3.1 | U1.7 15.51,15.64 15.62,15.75 15.62,16 | 15.62,16 15.62,16.14 | 15.62,16 15.49,16.13 | 15.76,16.14 15.62,16
  Top 0.406: C2.1 16.38,14.48 v16.26,14.35
  Bottom 0.406: v16.26,14.35 16,14.1 16,7.75 13.84,5.59 11.68,5.59 v11.56,5.71
  pour Top (isolate 0.254, no thermals): 15.62,16.13 15.62,14.15 15.8,13.97 16.38,13.97 16.64,14.22 16.64,16.13 16.51,16.26 15.75,16.26
  pour Top (isolate 0.254, no thermals): 11.94,4.7 11.94,6.73 11.43,7.24 10.41,7.24 9.14,8.51 7.99,8.51 7.63,8.14 7.65,6.98 9.4,5.33 10.67,5.33 11.43,4.57 11.81,4.57
VCC  (via drill 0.25 pad 0.51)
  Top 0.254: U1.5 13.7,14.43 13.84,14.29 14.1,14.29 | 14.2,14.74 U1.6 14.7,14.89 14.73,14.86 14.48,14.86 14.35,14.73 | 14.2,14.74 14.2,14.39 | 14.2,14.39 14.1,14.29 | 14.2,14.39 14.46,14.39 14.48,14.41 | 14.2,14.74 14.21,14.74 14.48,14.48 | 14.1,14.29 14.8,14.29
  Top 0.406: 14.48,14.41 14.67,14.41 | v5.33,15.11 R12.2 R13.2 | C4.1 15.11,13.97 14.67,14.41 | 14.67,14.41 v14.67,14.92 | R26.1 17.15,17.27 v17.27,17.4
  Bottom 0.406: v5.33,15.11 6.22,14.22 10.03,14.22 11.05,15.24 14.35,15.24 | v17.27,17.4 15.11,15.24 14.99,15.24 | 14.99,15.24 14.73,15.24 | 14.73,15.24 14.35,15.24 | v14.67,14.92 14.67,15.18 14.73,15.24 | v14.67,14.92 14.35,15.24 | v14.67,14.92 14.99,15.24

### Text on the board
tNames: GND | 3V3 | P0 | P6 | P1 | P7 | P2 | P8 | P3 | P9 | P4 | P10 | P5 | P11 | GND | P12 | RST | P13 | 3V3 | P14 | 5V | P15 | + | D- | P16 | - | RTC_PWR | D+ | P17 | GND | GND | RST | USR | RX | TX | PWR | USR
bNames: GND | 3V3 | P0 | P6 | P1 | P7 | P2 | P8 | P3 | P9 | P4 | P10 | P5 | P11 | GND | P12 | RST | P13 | 3V3 | P14 | 5V | P15 | D- | P16 | D+ | P17 | v1.0 | GND | GND

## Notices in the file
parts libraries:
SparkFun-Aesthetics: Licensing: Creative Commons ShareAlike 4.0 International - https://creativecommons.org/licenses/by-sa/4.0
moudle-new: This work is licensed under the Creative Commons Attribution 4.0 International License.
To view a copy of this license,visit: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
moudle-new: CC-BY-SA
